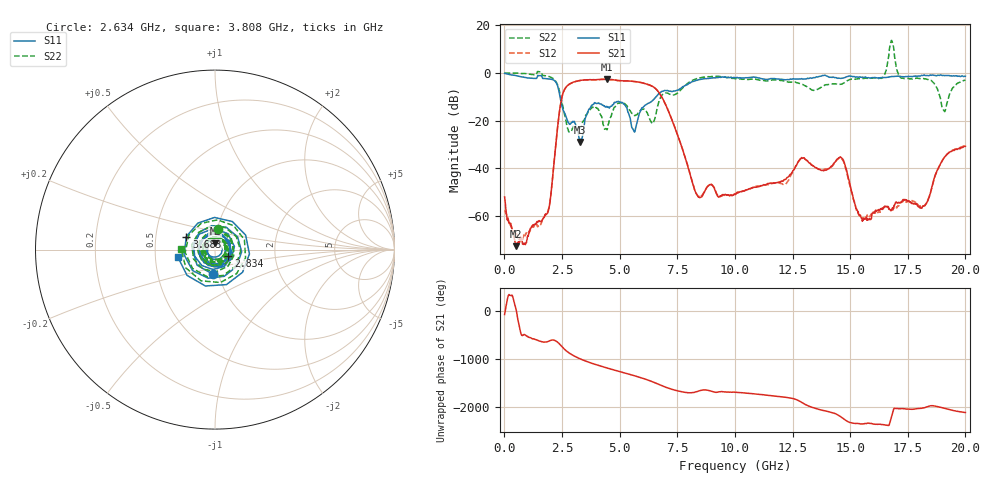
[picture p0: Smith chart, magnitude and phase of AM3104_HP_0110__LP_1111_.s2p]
!Created with skrf (http://scikit-rf.org).
# Hz S RI R 50.0
!freq ReS11 ImS11 ReS21 ImS21 ReS12 ImS12 ReS22 ImS22
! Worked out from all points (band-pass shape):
!   1601 points, 10 MHz to 20 GHz, reference 50 ohm
!   highest |S21| = -2.66 dB at 4.458 GHz (marker M1); lowest = -72.6 dB at 484.8 MHz (marker M2)
!   |S21| within 3 dB of the highest: 2.703 GHz to 6.433 GHz (3.73 GHz wide, 81.7 % of centre)
!   lowest |S11| = -29.0 dB at 3.283 GHz (marker M3), VSWR 1.07, Z = 50.1 + j3.56 ohm
!   |S11| at or under -10 dB: 2.414 GHz to 6.582 GHz (4.169 GHz wide, 92.7 % of centre)
!   |S22| runs from -24.8 to 13.6 dB; largest |S21 - S12| = 0.083
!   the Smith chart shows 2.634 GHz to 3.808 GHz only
!   S11 on the Smith chart (normalised r, x): 2.634 GHz: 0.94, -0.26; 2.834 GHz: 1.16, -0.09; 3.683 GHz: 0.72, +0.11; 3.808 GHz: 0.65, -0.05
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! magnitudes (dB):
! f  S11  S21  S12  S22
! 10 MHz  -0.2  -52.0  -57.6  -0.1
! 484.8 MHz  -1.1  -72.6  -67.2  -0.1
! 1.884 GHz  -2.5  -58.6  -58.0  -1.4
! 2.634 GHz  -17.2  -6.6  -6.5  -18.5
! 2.834 GHz  -21.6  -4.6  -4.7  -24.8
! 3.283 GHz  -29.0  -3.2  -3.2  -23.0
! 3.346 GHz  -27.7  -3.1  -3.1  -22.3
! 3.683 GHz  -15.1  -2.8  -2.9  -15.6
! 3.808 GHz  -13.5  -2.8  -2.8  -14.5
! 4.458 GHz  -14.1  -2.7  -2.7  -23.8
! 4.958 GHz  -11.9  -3.2  -3.2  -12.6
! 5.62 GHz  -24.4  -3.5  -3.6  -17.7
! 6.682 GHz  -8.9  -7.9  -7.9  -12.7
! 8.381 GHz  -3.0  -51.5  -51.3  -2.2
! 10.01 GHz  -2.0  -51.0  -50.7  -2.4
! 13.34 GHz  -2.2  -38.7  -38.7  -7.1
! 14.64 GHz  -2.2  -35.7  -36.1  -4.7
! 15.55 GHz  -1.8  -61.5  -60.9  -2.3
! 16.68 GHz  -1.7  -56.8  -56.9  7.3
! 18.19 GHz  -1.0  -55.8  -55.7  -2.4
! 19.06 GHz  -1.1  -35.7  -35.8  -15.8
! 20 GHz  -1.4  -30.8  -30.2  -3.0
